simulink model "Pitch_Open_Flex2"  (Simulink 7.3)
settings: Solver=ode4  StartTime=0.0  StopTime=20  RelTol=1e-3
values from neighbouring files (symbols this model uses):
  Apl = [    [plant.m]    (also in plant_z.m)
  Bpl = [    [plant.m]    (also in plant_z.m)
  Cpl = [    [plant.m]    (also in plant_z.m)
  Dpl = [    [plant.m]    (also in plant_z.m)
undefined symbols (not defined in the file or in its folder): Afc, Bfc, Cfc, Dfc

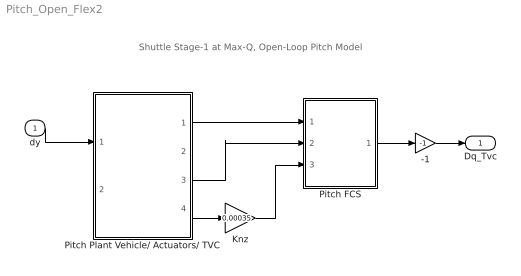
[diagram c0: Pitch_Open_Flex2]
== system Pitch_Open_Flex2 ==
  note: Shuttle Stage-1 at Max-Q, Open-Loop Pitch Model
  dy : Inport  OutDataType=sfix(16)  OutScaling=2^0
  -1 : Gain  Gain=-1  ParameterDataType=sfix(16)  ParameterScaling=2^0  OutDataType=sfix(16)  OutScaling=2^0
  Knz : Gain  Gain=0.00035  ParameterDataType=sfix(16)  ParameterScaling=2^0  OutDataType=sfix(16)  OutScaling=2^0
  Pitch FCS : Subsystem
  Pitch Plant Vehicle/ Actuators/ TVC : Subsystem
  Dq_Tvc : Outport  OutDataType=sfix(16)  OutScaling=2^0
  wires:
  dy/1 -> Pitch Plant Vehicle/ Actuators/ TVC/1(delt-c)
  Pitch Plant Vehicle/ Actuators/ TVC/1(theta) -> Pitch FCS/1(theta)
  Pitch Plant Vehicle/ Actuators/ TVC/4(Nz) -> Knz/1
  Knz/1 -> Pitch FCS/3(Nz)
  Pitch FCS/1(DQ_TVC) -> -1/1
  Pitch Plant Vehicle/ Actuators/ TVC/3(q-flx) -> Pitch FCS/2(q)
  -1/1 -> Dq_Tvc/1

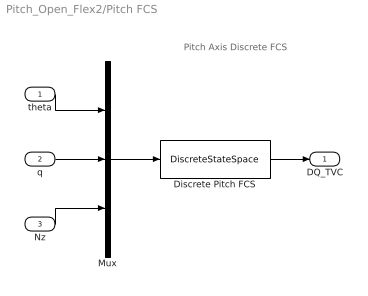
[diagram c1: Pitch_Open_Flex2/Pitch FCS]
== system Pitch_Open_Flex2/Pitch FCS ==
  note: Pitch Axis Discrete FCS
  theta : Inport  OutDataType=sfix(16)  OutScaling=2^0
  q : Inport  Port=2  OutDataType=sfix(16)  OutScaling=2^0
  Nz : Inport  Port=3  OutDataType=sfix(16)  OutScaling=2^0
  Discrete Pitch FCS : DiscreteStateSpace  A=Afc  B=Bfc  C=Cfc  D=Dfc  SampleTime=0.04
  Mux : Mux  Inputs=3
  DQ_TVC : Outport  OutDataType=sfix(16)  OutScaling=2^0
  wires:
  Discrete Pitch FCS/1 -> DQ_TVC/1
  theta/1 -> Mux/1
  q/1 -> Mux/2
  Nz/1 -> Mux/3
  Mux/1 -> Discrete Pitch FCS/1

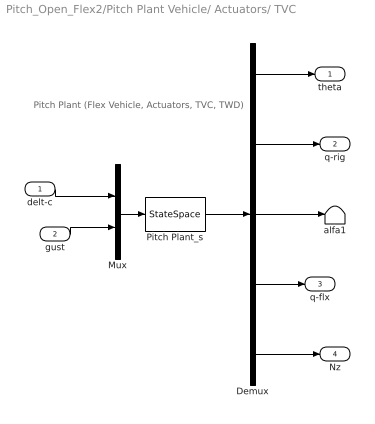
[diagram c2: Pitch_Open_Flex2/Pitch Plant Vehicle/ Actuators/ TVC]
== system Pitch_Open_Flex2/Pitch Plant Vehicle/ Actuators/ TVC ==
  note: Pitch Plant (Flex Vehicle, Actuators, TVC, TWD)
  delt-c : Inport  OutDataType=sfix(16)  OutScaling=2^0
  gust : Inport  Port=2  OutDataType=sfix(16)  OutScaling=2^0
  Demux : Demux  Outputs=5
  Mux : Mux  Inputs=2
  Pitch Plant_s : StateSpace  A=Apl  B=Bpl  C=Cpl  D=Dpl
  alfa1 : Terminator
  theta : Outport  OutDataType=sfix(16)  OutScaling=2^0
  q-rig : Outport  Port=2  OutDataType=sfix(16)  OutScaling=2^0
  q-flx : Outport  Port=3  OutDataType=sfix(16)  OutScaling=2^0
  Nz : Outport  Port=4  OutDataType=sfix(16)  OutScaling=2^0
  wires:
  Pitch Plant_s/1 -> Demux/1
  Mux/1 -> Pitch Plant_s/1
  delt-c/1 -> Mux/1
  gust/1 -> Mux/2
  Demux/1 -> theta/1
  Demux/3 -> alfa1/1
  Demux/4 -> q-flx/1
  Demux/2 -> q-rig/1
  Demux/5 -> Nz/1
